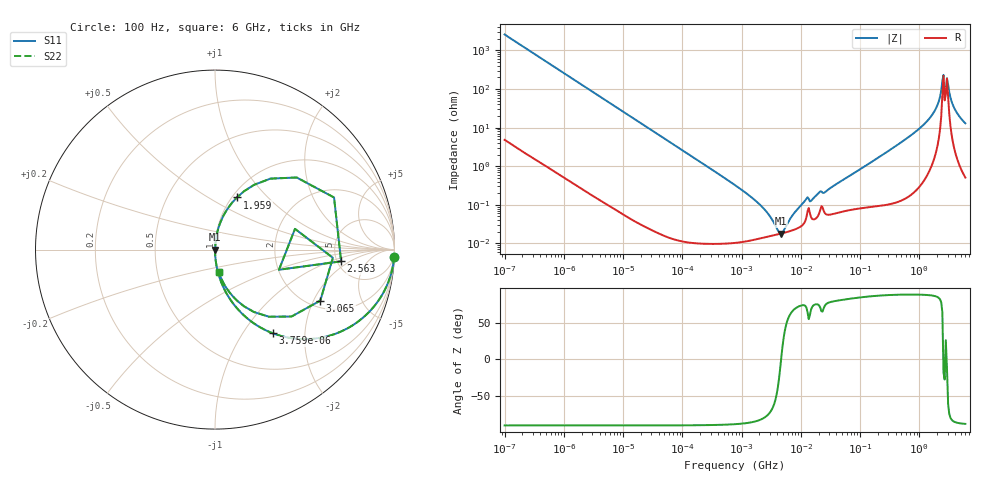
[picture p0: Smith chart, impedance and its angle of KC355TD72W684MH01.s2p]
!Murata Part Number: KC355TD72W684MH01
!These Parameters are Measured in Series Mode Connection
!Data Generated on Mar 13, 2026
!  o--ll--o
!Port1  Port2
!  o------o
!Operation Temp=25[degC], DC Bias Voltage=0[V]
!Freq. Start=100[Hz] Stop=6[GHz] 401[Steps]
# Hz S RI R 50
!Freq.(Hz) S11(Real) S11(Imag) S21(Real) S21(Imag) S12(Real) S12(Imag) S22(Real) S22(Imag)
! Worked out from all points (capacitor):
!   401 points, 100 Hz to 6 GHz, reference 50 ohm
!   read as one part in series: C = 617 nF near 109 Hz
!   lowest |Z| = 18.1 mohm at 4.644 MHz (marker M1)
!   series resonance near 4.646 MHz, so ESL is about 1.9 nH
!   S11 on the Smith chart (normalised r, x): 100 Hz: 1, -52; 3.759 kHz: 1.00, -1.38; 1.959 GHz: 1.05, +0.68; 2.563 GHz: 5.42, -1.41; 3.065 GHz: 2.28, -2.26; 6 GHz: 1.01, -0.26
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100  0.9984 -0.0387  0.00157 0.0387  0.00157 0.0387  0.9984 -0.0387
686  0.9338 -0.2477  0.0662 0.2477  0.0662 0.2477  0.9338 -0.2477
2008  0.6238 -0.4834  0.3762 0.4834  0.3762 0.4834  0.6238 -0.4834
3759  0.3222 -0.4663  0.6778 0.4663  0.6778 0.4663  0.3222 -0.4663
9204  0.074 -0.2607  0.926 0.2607  0.926 0.2607  0.074 -0.2607
40335  0.00431 -0.0641  0.9957 0.0641  0.9957 0.0641  0.00431 -0.0641
774597  0.000114 -0.00324  0.9999 0.00324  0.9999 0.00324  0.000114 -0.00324
2169299  0.000139 -0.000911  0.9999 0.000911  0.9999 0.000911  0.000139 -0.000911
4643984  0.000181 -4e-07  0.9998 4e-07  0.9998 4e-07  0.000181 -4e-07
1.189169e7  0.000384 0.00125  0.9996 -0.00125  0.9996 -0.00125  0.000384 0.00125
1.555665e7  0.000433 0.0013  0.9996 -0.0013  0.9996 -0.0013  0.000433 0.0013
2.035112e7  0.000597 0.002  0.9994 -0.002  0.9994 -0.002  0.000597 0.002
3.124326e8  0.0017 0.0257  0.9983 -0.0257  0.9983 -0.0257  0.0017 0.0257
1.094528e9  0.0145 0.1044  0.9855 -0.1044  0.9855 -0.1044  0.0145 0.1044
1.95892e9  0.1222 0.2906  0.8778 -0.2906  0.8778 -0.2906  0.1222 0.2906
2.240541e9  0.3086 0.3953  0.6914 -0.3953  0.6914 -0.3953  0.3086 0.3953
2.562649e9  0.7028 -0.0654  0.2972 0.0654  0.2972 0.0654  0.7028 -0.0654
2.679998e9  0.3565 -0.1122  0.6435 0.1122  0.6435 0.1122  0.3565 -0.1122
3.065283e9  0.5867 -0.2845  0.4133 0.2845  0.4133 0.2845  0.5867 -0.2845
3.352442e9  0.3006 -0.3741  0.6994 0.3741  0.6994 0.3741  0.3006 -0.3741
3.8344e9  0.1232 -0.2848  0.8768 0.2848  0.8768 0.2848  0.1232 -0.2848
6e9  0.0211 -0.1255  0.9789 0.1255  0.9789 0.1255  0.0211 -0.1255
